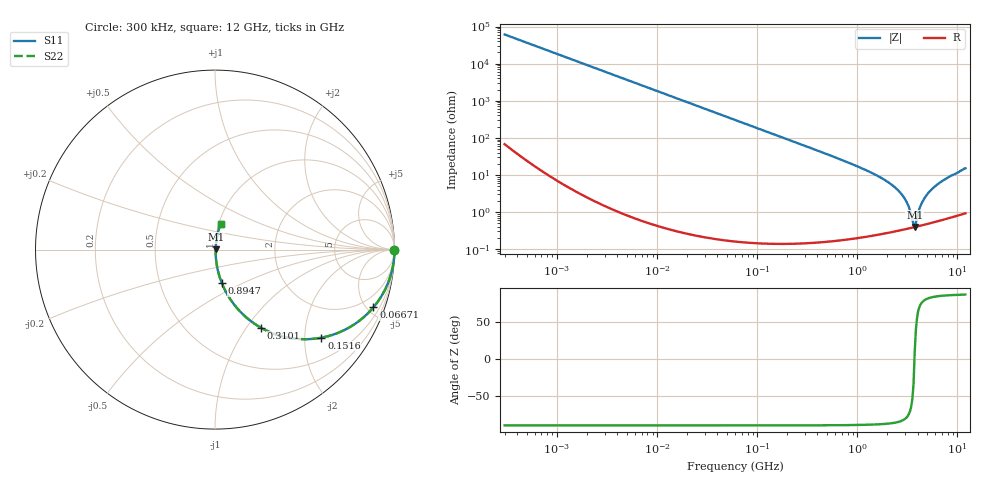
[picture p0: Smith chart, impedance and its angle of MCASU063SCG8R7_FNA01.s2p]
! MCASU063SCG8R7_FNA01  S-PARAMETER MODEL  ( General Type )
! Model Generated by TAIYO YUDEN Corporation (http://www.ty-top.com)
! Version 1.0
! TAIYO YUDEN Control No. 130801
! Copyright(c) 2013 TAIYO YUDEN CO.,LTD. All Rights Reserved.
! Product Description (link to TY-COMPAS)
! https://ds.yuden.co.jp/TYCOMPAS/or/detail?pn=MCASU063SCG8R7DFNA01&u=M
! Products Name : Multilayer Ceramic Capacitors
! Characteristics :
!  Capacitance : 8.7 pF , Rated Voltage : 50V , TCC : CG / C0G
!  Case Size : 0.6 x 0.3 / 0.024 x 0.012 [mm/inch] , Thickness : 0.3 / 0.012 [mm/inch]
!  (Conditions: Temperature = 25 degC , DC Bias Current/Voltage = 0A / 0V)
! External Node Assignments :
!  1  o---| |---o  2
! GND o---------o GND
! Frequency Range : 0.3MHz  -  12000MHz  [ 401 STEP ]
# MHz S RI R 50
! Freq[MHz].  S11 Real  S11 Imag  S21 Real  S21 Imag  S12 Real  S12 Imag  S22 Real  S22 Imag
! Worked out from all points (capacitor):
!   401 points, 300 kHz to 12 GHz, reference 50 ohm
!   read as one part in series: C = 8.68 pF near 316.3 kHz
!   lowest |Z| = 397 mohm at 3.741 GHz (marker M1)
!   series resonance near 3.722 GHz, so ESL is about 210 pH
!   S11 on the Smith chart (normalised r, x): 300 kHz: open; 66.71 MHz: 1.00, -5.50; 151.6 MHz: 1.00, -2.41; 310.1 MHz: 1.00, -1.17; 894.7 MHz: 1.00, -0.39; 12 GHz: 1.02, +0.30
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0.3  1 -0.00164  4.48e-06 0.00164  4.48e-06 0.00164  1 -0.00164
1.769972  0.9999 -0.00965  9.59e-05 0.00965  9.59e-05 0.00965  0.9999 -0.00965
10.44266  0.9968 -0.0568  0.00325 0.0568  0.00325 0.0568  0.9968 -0.0568
26.39317  0.9797 -0.141  0.0203 0.141  0.0203 0.141  0.9797 -0.141
60  0.9031 -0.2956  0.0969 0.2956  0.0969 0.2956  0.9031 -0.2956
66.70707  0.8829 -0.3213  0.1171 0.3213  0.1171 0.3213  0.8829 -0.3213
151.6462  0.5929 -0.4907  0.4071 0.4907  0.4071 0.4907  0.5929 -0.4907
310.0777  0.2569 -0.4357  0.7431 0.4357  0.7431 0.4357  0.2569 -0.4357
353.9943  0.2092 -0.4053  0.7908 0.4053  0.7908 0.4053  0.2092 -0.4053
894.6982  0.0377 -0.1856  0.9623 0.1856  0.9623 0.1856  0.0377 -0.1856
2088.533  0.00638 -0.0598  0.9936 0.0598  0.9936 0.0598  0.00638 -0.0598
2514.07  0.00465 -0.0397  0.9953 0.0397  0.9953 0.0397  0.00465 -0.0397
2947.191  0.00392 -0.0234  0.9961 0.0234  0.9961 0.0234  0.00392 -0.0234
3276.641  0.00376 -0.0129  0.9962 0.0129  0.9962 0.0129  0.00376 -0.0129
3547.679  0.00381 -0.00512  0.9962 0.00512  0.9962 0.00512  0.00381 -0.00512
3740.715  0.00391 0.000622  0.9961 -0.000622  0.9961 -0.000622  0.00391 0.000622
3841.137  0.00399 0.00315  0.996 -0.00315  0.996 -0.00315  0.00399 0.00315
4270.516  0.00445 0.0137  0.9956 -0.0137  0.9956 -0.0137  0.00445 0.0137
4502.883  0.00478 0.019  0.9952 -0.019  0.9952 -0.019  0.00478 0.019
5420.343  0.00646 0.0379  0.9935 -0.0379  0.9935 -0.0379  0.00646 0.0379
7448.838  0.0118 0.0738  0.9882 -0.0738  0.9882 -0.0738  0.0118 0.0738
12000  0.0307 0.1447  0.9693 -0.1447  0.9693 -0.1447  0.0307 0.1447
